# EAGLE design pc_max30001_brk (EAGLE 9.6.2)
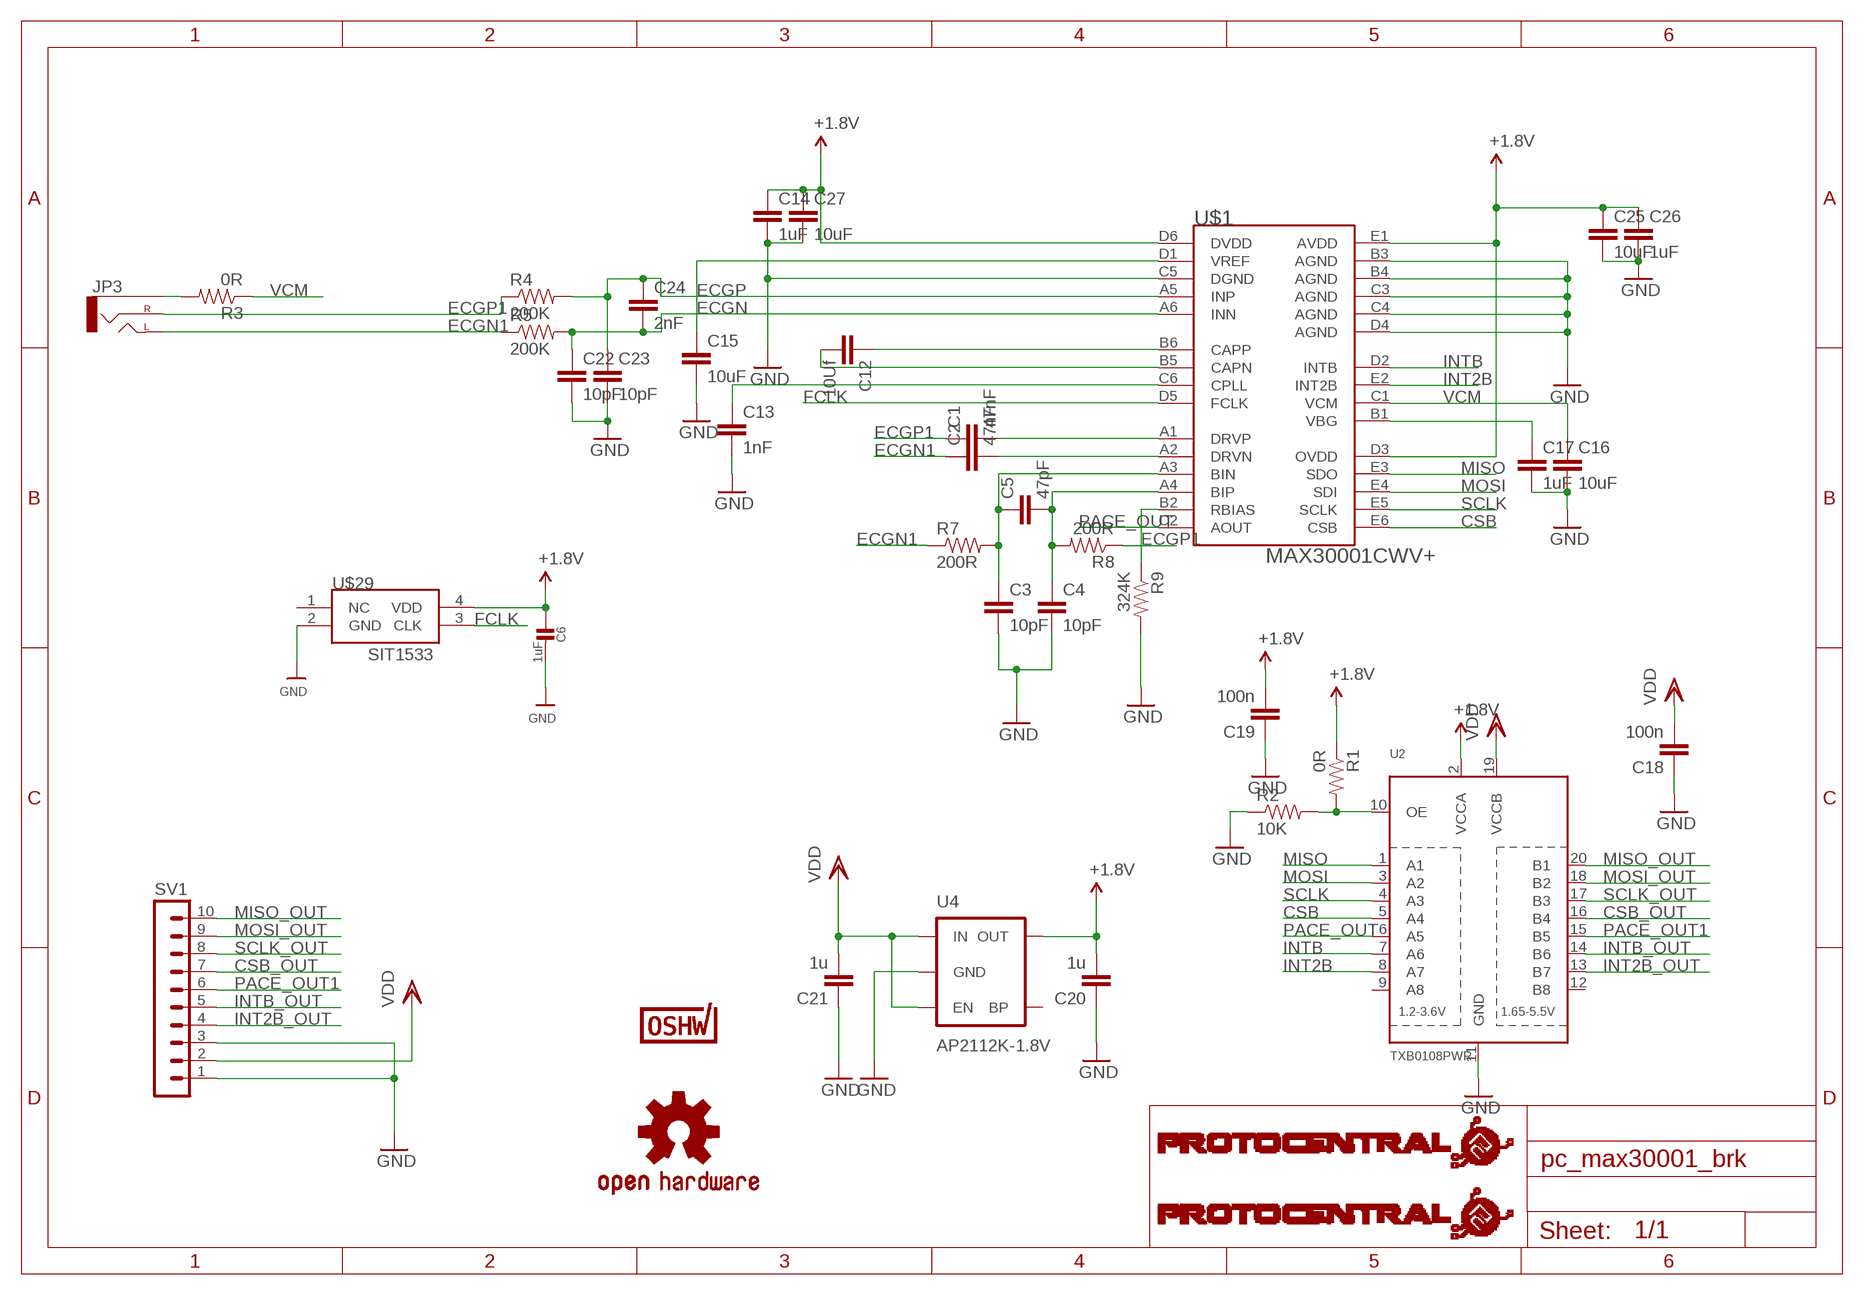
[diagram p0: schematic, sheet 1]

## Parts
C1  47nF  C-EUC0402  [C0402]
C2  47nF  C-EUC0402  [C0402]
C3  10pF  C-EUC0402  [C0402]
C4  10pF  C-EUC0402  [C0402]
C5  47pF  C-EUC0402  [C0402]
C6  1uF  CAP_CERAMIC0402  [0402]
C12  10Uf  C-EUC0805  [C0805]
C13  1nF  C-EUC0402  [C0402]
C14  1uF  C-EUC0402  [C0402]
C15  10uF  C-EUC0805  [C0805]
C16  10uF  C-EUC0805  [C0805]
C17  1uF  C-EUC0402  [C0402]
C18  100n  C-EUC0402  [C0402]
C19  100n  C-EUC0402  [C0402]
C20  1u  C-EUC0805  [C0805]
C21  1u  C-EUC0805  [C0805]
C22  10pF  C-EUC0402  [C0402]
C23  10pF  C-EUC0402  [C0402]
C24  2nF  C-EUC0402  [C0402]
C25  10uF  C-EUC0805  [C0805]
C26  1uF  C-EUC0402  [C0402]
C27  10uF  C-EUC0805  [C0805]
JP3  AUDIO-JACKSMD2  [AUDIO-JACK-3.5MM-SMD]
R1  0R  RESISTOR0805-RES  [0805]
R2  10K  RESISTOR0805-RES  [0805]
R3  0R  RESISTOR0805-RES  [0805]
R4  200K  RESISTOR0805-RES  [0805]
R5  200K  RESISTOR0805-RES  [0805]
R7  200R  RESISTOR0402-RES  [0402-RES]
R8  200R  RESISTOR0402-RES  [0402-RES]
R9  324K  RESISTOR0402-RES  [0402-RES]
SV1  MA10-1  [MA10-1]
U2  TXB0108PWR  [TSSOP20]
U4  AP2112K-1.8V  V_REG_LDOSMD  [SOT23-5]
U$1  MAX30001CWV+  [30WLP]
U$3  PROTY-LOGO  [LOGO-PROTY]
U$4  PROTY_LOGO_WITH_TEXT  [PROTY_WITH_TEXT]
U$6  OSHW-LOGOS  [OSHW-LOGO-S]
U$7  CERT-SMALL  [CERT-SMALL-SILK]
U$29  SIT1533  [SIT1533]

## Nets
+1.8V: C6.1 C14.1 C19.2 C20.2 C25.1 C26.1 C27.1 R1.1 U2.2(VCCA) U4.5(OUT) U$1.D3(OVDD) U$1.D6(DVDD) U$1.E1(AVDD) U$29.4(VDD)
CSB: U2.5(A4) U$1.E6(CSB)
CSB_OUT: SV1.7 U2.16(B4)
ECGN: C22.1 C24.2 R5.2 U$1.A6(INN)
ECGN1: C2.1 JP3.TIP(LEFT) R5.1 R7.1
ECGP: C23.1 C24.1 R4.2 U$1.A5(INP)
ECGP1: C1.1 JP3.RING(RIGHT) R4.1 R8.1
FCLK: U$1.D5(FCLK) U$29.3(CLK)
GND: C3.2 C4.2 C6.2 C13.2 C14.2 C15.2 C16.2 C17.2 C18.1 C19.1 C20.1 C21.1 C22.2 C23.2 C25.2 C26.2 C27.2 R2.1 R9.2 SV1.1 SV1.3 U2.11(GND) U4.2(GND) U$1.B3(AGND) U$1.B4(AGND) U$1.C3(AGND) U$1.C4(AGND) U$1.C5(DGND) U$1.D4(AGND) U$29.2(GND)
INT2B: U2.8(A7) U$1.E2(INT2B)
INT2B_OUT: SV1.4 U2.13(B7)
INTB: U2.7(A6) U$1.D2(INTB)
INTB_OUT: SV1.5 U2.14(B6)
MISO: U2.1(A1) U$1.E3(SDO)
MISO_OUT: SV1.10 U2.20(B1)
MOSI: U2.3(A2) U$1.E4(SDI)
MOSI_OUT: SV1.9 U2.18(B2)
N$1: C12.1 U$1.B6(CAPP)
N$2: C1.2 U$1.A1(DRVP)
N$4: C2.2 U$1.A2(DRVN)
N$5: C3.1 C5.1 R7.2 U$1.A3(BIN)
N$6: C4.1 C5.2 R8.2 U$1.A4(BIP)
N$7: R9.1 U$1.B2(RBIAS)
N$10: C13.1 U$1.C6(CPLL)
N$12: C12.2 U$1.B5(CAPN)
N$13: C15.1 U$1.D1(VREF)
N$15: C17.1 U$1.B1(VBG)
N$16: R1.2 R2.2 U2.10(OE)
N$19: JP3.SLEEVE R3.2
PACE_OUT: U2.6(A5) U$1.C2(AOUT)
PACE_OUT1: SV1.6 U2.15(B5)
SCLK: U2.4(A3) U$1.E5(SCLK)
SCLK_OUT: SV1.8 U2.17(B3)
VCM: C16.1 R3.1 U$1.C1(VCM)
VDD: C18.2 C21.2 SV1.2 U2.19(VCCB) U4.1(IN) U4.3(EN)
Unconnected: U2.9(A8) U2.12(B8) U4.4(BP) U$29.1(NC)

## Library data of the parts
C1-C5 C12-C27 = rcl:C-EU: CAPACITOR, European symbol; SPICEPREFIX: C
C6 = microbuilder:CAP_CERAMIC: Ceramic Capacitors
JP3 = SparkFun-Connectors:AUDIO-JACK: 3.5mm Audio Jack Simple 3.5mm common PCB mount audio jack. SKU: PRT-08032; PROD_ID: CONN-10353
R1-R5 R7-R9 = SparkFun:RESISTOR: Resistor
SV1 = con-lstb:MA10-1: PIN HEADER; OC_FARNELL: unknown; OC_NEWARK: unknown
U2 = adafruit:TXB0108PWR: 8-Bit Bi-Directional Level Shifter 1.2V-3.6V (VCCA) to 1.65V-5.5V (VCCB) bi-directional level shifter with auto direction sensing. Max data rate - VCCA 1.8V: 20Mbps (50ns), VCCA 3.3V: 100Mbps (10ns) Digikey: 296-21527-1-ND
U4 = SparkFun-PowerIC:V_REG_LDO: Voltage Regulator LDO Standard 150mA LDO voltage regulator in SOT-23 layout. Micrel part MIC5205. BP (by-pass) pin is used to lower output noise with 470pF cap.; PROD_ID: VREG-12457
U$1 = circuitects:MAX30001CWV+
U$3 = circuitects:PROTY-LOGO
U$4 = circuitects:PROTY_LOGO_WITH_TEXT
U$6 = SparkFun:OSHW-LOGO: Open Source Hardware Logo This logo indicates the piece of hardware it is found on incorporates a OSHW license and/or adheres to the definition of open source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
U$7 = OSHWA:CERT
U$29 = circuitects:SIT1533

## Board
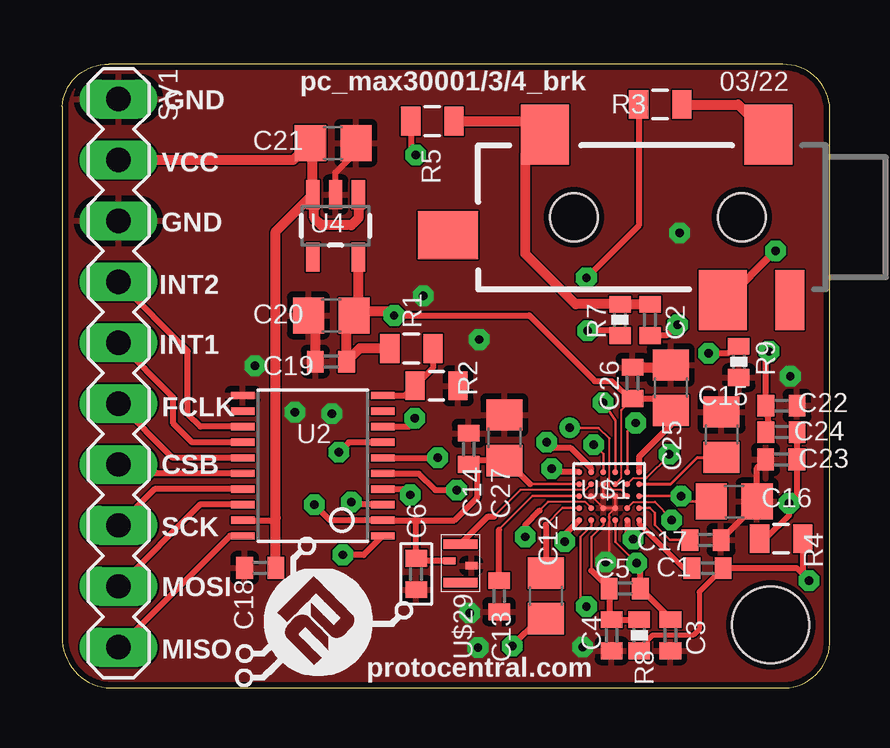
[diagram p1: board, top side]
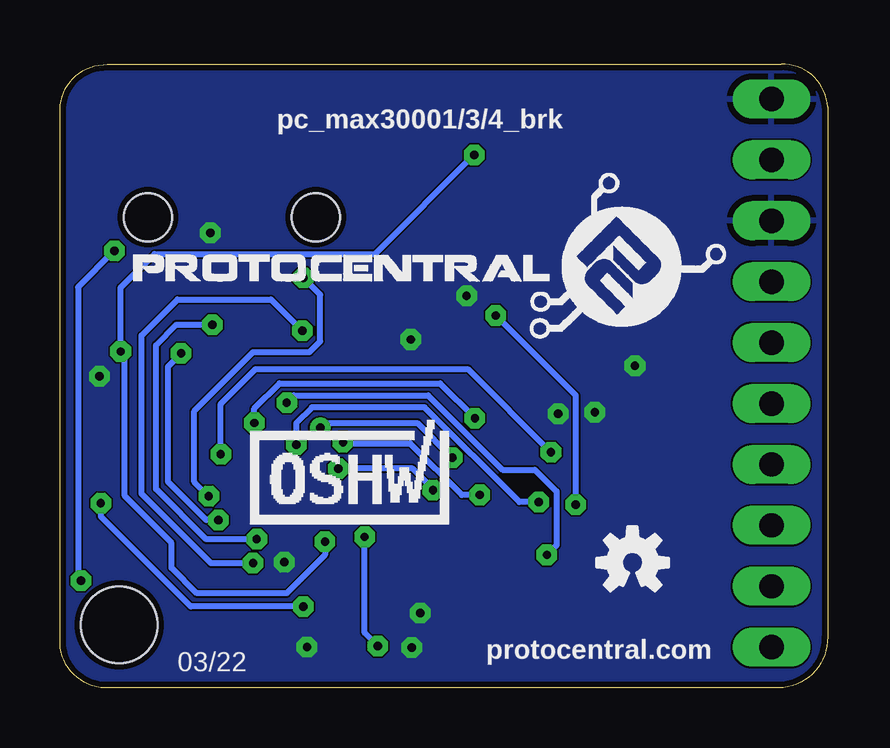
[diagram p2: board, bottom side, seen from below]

Size 32 x 26 mm. Coordinates in mm from the lower left corner, seen from the top.
Outline: 2.03,0 30.13,0 arc90 32,2.03 32,24.13 arc90 30.03,26 1.93,26 arc90 0,24.23 0,2.13 arc90 2.03,0
Copper layers (1*2*15*16): Top 0.035mm / dielectric 1.5mm / Route2 0.035mm / dielectric 0.15mm / Route15 0.035mm / dielectric 0.2mm / Bottom 0.035mm
Design rules "Circuitects-Rules *": minimum track width 2mil, minimum drill 0.05mm, track to track 0.06858125mm, track to pad 0.06858125mm, pad to pad 0.06858125mm, via to via 4mil, smd to smd 4mil, copper to edge 10mil, drill to drill 8mil, minimum pad ring 12mil, minimum via ring 10mil, stop-mask expansion 4mil, vias tented up to drill 25mil, thermal gap 10mil
Holes 3.2 mm at 29.53,2.63

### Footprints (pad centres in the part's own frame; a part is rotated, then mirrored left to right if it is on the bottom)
C0402 = smd 0.7 x 0.9: 1 -0.65,0; 2 0.65,0
0402 = smd 0.7 x 0.9: 1 -0.65,0; 2 0.65,0
C0805 = smd 1.3 x 1.5: 1 -0.95,0; 2 0.95,0
AUDIO-JACK-3.5MM-SMD = smd 2 x 2.5: RING 4.3,3.45; SLEEVE 2.4,-3.45; TIP 11.7,-3.45 | smd 1.2 x 2.5: RSH 1.5,3.45 | smd 2.5 x 2: TSH 15.75,0.75 | hole 2: 3.5,0; 10.5,0
0805 = smd 0.8 x 1.2: 1 -0.9,0; 2 0.9,0
0402-RES = smd 0.7 x 0.9: 1 -0.65,0; 2 0.65,0
MA10-1 = drill 1.016 long: 1 -11.43,0; 2 -8.89,0; 3 -6.35,0; 4 -3.81,0; 5 -1.27,0; 6 1.27,0; 7 3.81,0; 8 6.35,0; 9 8.89,0; 10 11.43,0
TSSOP20 = smd 0.305 x 0.991: 1 -2.925,-2.918; 2 -2.275,-2.918; 3 -1.625,-2.918; 4 -0.975,-2.918; 5 -0.325,-2.918; 6 0.325,-2.918; 7 0.975,-2.918; 8 1.625,-2.918; 9 2.275,-2.918; 10 2.925,-2.918; 11 2.925,2.918; 12 2.275,2.918; 13 1.625,2.918; 14 0.975,2.918; 15 0.325,2.918; 16 -0.325,2.918; 17 -0.975,2.918; 18 -1.625,2.918; 19 -2.275,2.918; 20 -2.925,2.918
SOT23-5 = smd 0.55 x 1.2: 1 -0.95,-1.3; 2 0,-1.3; 3 0.95,-1.3; 4 0.95,1.3; 5 -0.95,1.3
30WLP = smd 0.25 x 0.25: A1 -1.25,1; A2 -0.75,1; A3 -0.25,1; A4 0.25,1; A5 0.75,1; A6 1.25,1; B1 -1.25,0.5; B2 -0.75,0.5; B3 -0.25,0.5; B4 0.25,0.5; B5 0.75,0.5; B6 1.25,0.5; C1 -1.25,0; C2 -0.75,0; C3 -0.25,0; C4 0.25,0; C5 0.75,0; C6 1.25,0; D1 -1.25,-0.5; D2 -0.75,-0.5; D3 -0.25,-0.5; D4 0.25,-0.5; D5 0.75,-0.5; D6 1.25,-0.5; E1 -1.25,-1; E2 -0.75,-1; E3 -0.25,-1; E4 0.25,-1; E5 0.75,-1; E6 1.25,-1
SIT1533 = smd 0.4 x 1.4: 1 -0.8,0; 3 0.8,0 | smd 0.3 x 0.5: 2 -0.1,-0.45; 4 0.1,0.45

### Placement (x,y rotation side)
C1  26.9,5 180 top
C2  24.5,15.35 270 top
C3  25.35,2.2 270 top
C4  22.9,2.2 270 top
C5  23.45,4.15 180 top
C6  14.75,4.75 270 top
C12  20.16,3.84 270 top
C13  18.21,3.83 270 top
C14  16.94,9.97 90 top
C15  27.48,10.56 90 top
C16  28.01,7.77 0 top
C17  26.81,6.17 0 top
C18  8.25,5.01 0 top
C19  11.2,13.61 0 top
C20  11.21,15.53 0 top
C21  11.29,22.72 180 top
C22  29.98,11.77 0 top
C23  29.97,9.53 180 top
C24  29.98,10.67 180 top
C25  25.37,12.52 90 top
C26  23.77,12.72 90 top
C27  18.43,10.43 90 top
JP3  31.83,19.63 180 top
R1  14.55,14.16 0 top
R2  15.6,12.6 180 top
R3  24.93,24.33 0 top
R4  29.97,6.23 180 top
R5  15.43,23.63 180 top
R7  23.25,15.35 270 top
R8  24.05,2.2 90 top
R9  28.2,13.6 270 top
SV1  2.34,13.13 270 top
U2  10.44,9.27 90 top
U4  11.39,19.27 180 top
U$1  22.8,8 180 top
U$3  7.13,-0.07 0 top
U$4  28.93,14.93 0 bottom
U$6  8.13,5.23 0 bottom
U$7  19.93,6.83 0 bottom
U$29  16.6,5.2 90 top

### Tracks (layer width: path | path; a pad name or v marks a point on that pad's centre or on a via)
+1.8V  (via drill 0.35)
  Top 0.076: U$1.D3 23.3,8.75 23.3,11.6
  Top 0.102: U$1.D6 19.5,8.5 | 23.3,11.6 23.7,12 C26.1
  Top 0.254: 19.5,8.5 18.52,9.48 C27.1 | C27.1 17.1,9.48 C14.1 17.3,8.96 17.3,7.95 16.34,7 14.7,7 | C27.1 18.93,9.48 | v13.83,15.53 19.47,15.53 22.2,12.8 22.9,12.8 23.7,12 | C26.1 24.87,12.07 C25.1 25.37,10.97 24.05,9.65 U$1.E1 | v10.5,7.65 11.15,7 U2.2 14.7,7 | U$29.4 14.85,5.3 C6.1 14.75,6.95 14.7,7
  Top 0.406: R1.1 12.4,14.16 C19.2 11.85,15.22 C20.2 12.34,15.71 | 12.34,15.71 13.65,15.71 v13.83,15.53 | 12.34,15.71 U4.5
  Bottom 0.254: v10.5,7.65 10.5,12.2 v13.83,15.53
CSB  (via drill 0.35)
  Top 0.254: U2.5 14.86,8.95 15.55,8.25 v16.45,8.25 | U$1.E6 20.55,9 v20.4,9.15
  Bottom 0.254: v16.45,8.25 16.45,8.3 17.3,9.15 v20.4,9.15
CSB_OUT
  Top 0.254: U2.16 2.71,8.95 SV1.7
ECGN  (via drill 0.35)
  Top 0.254: R5.2 14.53,22.43 v14.73,22.23 | U$1.A6 20.95,6.4 v20.95,6.1 | C24.2 29.47,10.81 C22.1 29.33,13.89 v29.47,14.03
  Bottom 0.254: v14.73,22.22 v14.73,22.23 18.86,18.1 28.06,18.1 29.47,16.69 v29.47,14.03 29.3,13.86 29.3,8 27.35,6.05 27.35,5 26.3,3.95 22.55,3.95 20.95,5.55 v20.95,6.1
ECGN1
  Top 0.406: R5.1 19.58,23.63 JP3.TIP 19.3,22.25 19.3,18.1 21.4,16 R7.1 C2.1
ECGP  (via drill 0.35)
  Top 0.102: U$1.A5 22.05,6.75 21.6,6.3 21.6,3.65 v21.85,3.4
  Top 0.254: C24.1 C23.1 30.62,8.02 v30.3,7.7 30.3,7.2 29.33,6.23 R4.2
  Bottom 0.254: v21.85,3.4 26.55,3.4 30.3,7.15 v30.3,7.7
ECGP1  (via drill 0.35)
  Top 0.2: C1.1 26.55,4 26.55,2.45 26.3,2.2 24.6,2.2 24.05,1.65 R8.1
  Top 0.254: R8.1 24.2,1.7 | 27.4,4.85 C1.1 30.61,5 v31.13,4.48 30.87,4.74 R4.1
  Top 0.305: JP3.RING 27.68,16.18 v29.73,18.23
  Bottom 0.254: v29.73,18.23 31.25,16.71 31.25,4.6 v31.13,4.48
FCLK
  Top 0.076: U$1.D5 21.8,8.25 19.1,8.25
  Top 0.102: 18,7.15 19.1,8.25
  Top 0.254: U$29.3 17.75,7.15 18,7.15
GND  (via drill 0.35)
  Top 0.076: U$1.B3 22.8,7.25 22.8,5.4
  Top 0.102: U$1.D4 U$1.C4 U$1.C3 U$1.B3 | U$1.C5 U$1.B4
  Top 0.134: U$1.B4 U$1.B3
  Top 0.254: U4.2 11.39,21.49 12.24,22.34 C21.1 | C17.2 28.96,7.67 C16.2 28.96,9.17 C23.2 | v22.65,5.25 22.8,5.4
  Top 0.406: C19.1 10.55,15.24 C20.1 | R9.2 28.17,13.08 | C26.2 25.27,13.37 C25.2
  other vias: 8.03,13.43 17.33,1.68 16.98,3.13 11.23,11.43 25.73,18.98 17.38,14.53 15.05,16.35 21.7,1.7 9.7,11.5 30.35,13
  pour Top: 0,26.33 32,26.33 32,0 0,0
  pour Bottom: 0,26 32,26 32,0 0,0
INT2B  (via drill 0.35)
  Top 0.102: U$1.E2 23.55,10.7 v23.9,11.05
  Top 0.254: U2.8 14.45,10.89 v14.7,11.25
  Bottom 0.254: v23.9,11.05 23.9,11.65 22.85,12.7 16.15,12.7 v14.7,11.25
INT2B_OUT
  Top 0.254: U2.13 5.76,10.89 5.23,11.43 5.23,14.05 SV1.4
INTB  (via drill 0.35)
  Top 0.076: U$1.D2 23.8,8.75 24.35,8.75
  Top 0.102: v25.3,9.75 25.3,9.7 24.35,8.75
  Top 0.254: U2.7 11.95,10.24 v11.53,9.83
  Bottom 0.254: v11.53,9.83 15,13.3 23.85,13.3 25.3,11.85 v25.3,9.75
INTB_OUT
  Top 0.254: U2.14 5.42,10.24 4.63,11.03 4.63,12.11 SV1.5
MISO  (via drill 0.35)
  Top 0.102: v22.55,11.9 23.05,11.15 U$1.E3
  Top 0.254: U2.1 12.56,5.55 v11.7,5.55
  Bottom 0.254: v22.55,11.9 22.25,12.2 16.65,12.2 13.55,9.1 12.2,9.1 11.3,8.2 11.3,5.95 v11.7,5.55
MISO_OUT
  Top 0.254: U2.20 6.99,6.34 SV1.10
MOSI  (via drill 0.35)
  Top 0.102: v22.15,10.15 22.55,9.75 U$1.E4
  Top 0.254: U2.3 12.15,7.64 v12.05,7.75
  Bottom 0.254: v12.05,7.75 12.85,7.75 16.8,11.7 21.5,11.7 22.15,11.05 v22.15,10.15
MOSI_OUT
  Top 0.254: U2.18 5.75,7.64 SV1.9
N$1
  Top 0.102: U$1.B6 20.85,7.5 20.16,6.81
  Top 0.254: 20.16,6.81 C12.1
N$2
  Top 0.2: U$1.A1 24.05,6.85 25.9,5 C1.2
N$4  (via drill 0.35)
  Top 0.254: U$1.A2 23.55,6.45 v23.8,6.2 | v25.65,15.15 25.2,14.7 C2.2
  Bottom 0.254: v23.8,6.2 25.9,6.2 28,8.3 28,14.3 27.15,15.15 v25.65,15.15
N$5  (via drill 0.35)
  Top 0.102: U$1.A3 23.05,6.1 v23.95,5.2
  Top 0.254: C3.1 25.35,2.9 C5.1 24.1,5.05 v23.95,5.2 | R7.2 23.05,14.9 v21.9,14.9
  Bottom 0.254: v23.95,5.2 25.7,5.2 28.6,8.1 28.6,14.7 27.1,16.2 23.2,16.2 v21.9,14.9
N$6
  Top 0.102: U$1.A4 22.55,6.8 22.05,6.3 22.05,4.9
  Top 0.254: 22.05,4.9 C5.2 22.8,2.95 C4.1 R8.2
N$7  (via drill 0.35)
  Top 0.076: U$1.B2 23.8,7.75 24.7,7.75
  Top 0.1: U$1.B2 23.6,7.5
  Top 0.102: v25.4,7 25.4,7.05 24.7,7.75
  Top 0.254: R9.1 27.75,13.95 v26.95,13.95
  Bottom 0.254: v25.4,7 25.9,7 27.5,8.6 27.5,13.4 v26.95,13.95
N$10
  Top 0.102: 18.21,6.61 19.6,8 U$1.C6
  Top 0.254: C13.1 18.21,6.61
N$12  (via drill 0.35)
  Top 0.076: U$1.B5 21.8,7.75 20.25,7.75
  Top 0.102: 20.25,7.75 19.9,7.4
  Top 0.254: C12.2 19.89,2.89 v18.75,1.75 | 19.9,7.4 19.3,6.8 v19.3,6.3
  Bottom 0.254: v19.3,6.3 19.3,2.3 v18.75,1.75
N$13
  Top 0.127: U$1.D1 25.37,8.5 26.48,9.61 C15.1
N$15
  Top 0.102: C17.1 25.33,6.17 24.7,6.8 24.7,7.3 24.5,7.5 U$1.B1
N$16
  Top 0.254: U2.10 14.29,12.2 R2.2 15.45,13.35 R1.2
N$19
  Top 0.406: R3.2 28.18,24.33 JP3.SLEEVE
PACE_OUT  (via drill 0.35)
  Top 0.076: U$1.C2 23.3,8.25 22.95,8.25 22.8,8.4 22.8,10.4
  Top 0.102: 22.8,10.4 22.35,10.85 v21.15,10.85
  Top 0.254: U2.6 v15.64,9.6 v15.65,9.6
  Bottom 0.254: v21.15,10.85 20.95,11.05 17.1,11.05 v15.65,9.6
PACE_OUT1
  Top 0.254: U2.15 4.61,9.6 SV1.6
SCLK  (via drill 0.35)
  Top 0.102: U$1.E5 22.05,9.15
  Top 0.254: U2.4 14.26,8.29 v14.5,8.05 | v20.2,10.25 20.45,10 21.2,10 22.05,9.15
  Bottom 0.254: v20.2,10.25 19.85,10.2 17.4,10.2 15.25,8.05 v14.5,8.05
SCLK_OUT
  Top 0.254: U2.17 3.85,8.29 SV1.8
VCM  (via drill 0.35)
  Top 0.102: U$1.C1 v25.8,8 26.03,7.77 C16.1
  Top 0.254: R3.1 24.03,19.28 v21.85,17.1
  Bottom 0.254: v25.8,8 26.4,8.6 26.4,11.55 23.95,14 21.6,14 21.15,14.45 21.15,16.4 v21.85,17.1
VDD
  Top 0.254: U2.19 8.79,7 8.9,7.1
  Top 0.406: U4.3 10.44,22.62 C21.2 9.64,22.02 SV1.2 | C18.2 8.9,7.1 8.9,19.03 U4.3 | U4.1 12.34,19.59 12.05,19.3 10.8,19.3 10.5,19.6 10.5,20.51 U4.3

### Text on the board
tPlace: pc_max30001/3/4_brk | 03/22 | GND | VCC | GND | INT2 | INT1 | FCLK | CSB | SCK | MOSI | MISO | protocentral.com
bPlace: pc_max30001/3/4_brk | protocentral.com | 03/22

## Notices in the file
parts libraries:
SparkFun-PowerIC: Licensing: Creative Commons ShareAlike 4.0 International - https://creativecommons.org/licenses/by-sa/4.0
microbuilder: This work is placed in the public domain, and may be freely used for commercial and non-commercial work with the following conditions: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
